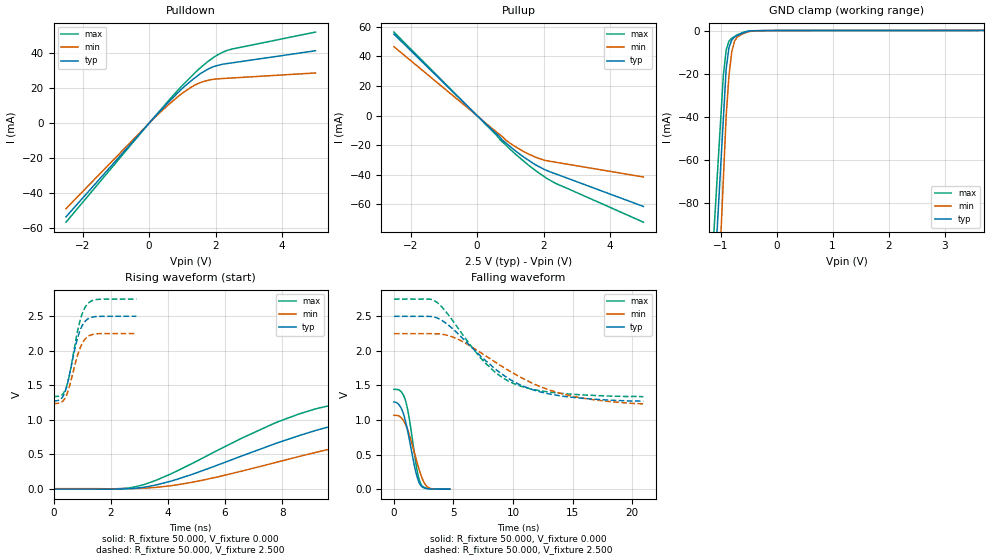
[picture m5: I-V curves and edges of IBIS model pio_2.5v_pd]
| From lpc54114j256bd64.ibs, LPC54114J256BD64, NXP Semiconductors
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[Model]   pio_2.5v_pd
Model_type I/O
Vinl=4.000E-01
Vinh=1.500E+00
Vref=0.000E+00
Rref=1.000E+06
Cref=2.000E-11
Vmeas=1.250E+00
C_comp   9.060E-12   8.700E-12   9.420E-12
[Voltage Range]   2.500E+00   2.250E+00   2.750E+00
[POWER Clamp Reference]   2.500E+00   2.250E+00   2.750E+00
[GND Clamp Reference]   0.000E+00   0.000E+00   0.000E+00
[Pullup Reference]   2.500E+00   2.250E+00   2.750E+00
[Pulldown Reference]   0.000E+00   0.000E+00   0.000E+00
[Temperature Range]   25   105   -40
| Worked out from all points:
|   slope of the pulldown table from 0 to 0.375 V, typ, clamps not added: 48.2 ohm
|   slope of the pullup table from 0 to 0.375 V, typ, clamps not added: 47.2 ohm
|   GND clamp passes 1 mA (typ) near -0.58 V on its own axis
|   rising waveform, R_fixture 50.000, V_fixture 0.000: 20-80 % time 5.59ns typ, 6.98ns min, 4.66ns max; typ from -0.006 V to 1.26 V
|   falling waveform, R_fixture 50.000, V_fixture 0.000: 20-80 % time 902ps typ, 1.09ns min, 781ps max; typ from 1.26 V to 0 V
|   rising waveform, R_fixture 50.000, V_fixture 2.500: 20-80 % time 408ps typ, 413ps min, 407ps max; typ from 1.27 V to 2.5 V
|   falling waveform, R_fixture 50.000, V_fixture 2.500: 20-80 % time 5.14ns typ, 6.37ns min, 4.26ns max; typ from 2.5 V to 1.27 V
[GND Clamp]
-2.5V     -757.5mA   -973.5mA   -687.5mA
-950mV    -40.89mA   -68.88mA   -20.67mA
-900mV    -17.78mA   -39.7mA    -9.038mA
-850mV    -7.888mA   -20.93mA   -4.915mA
-800mV    -4.357mA   -9.856mA   -3.541mA
-750mV    -3.031mA   -4.855mA   -2.756mA
-700mV    -2.227mA   -2.959mA   -1.97mA
-600mV    -1.164mA   -1.43mA    -872.3uA
-500mV    -329.3uA   -546.9uA   -245.1uA
-200mV    -21.96uA   -28.58uA   -10.55uA
5V        98.58uA    104.9uA    95.1uA
[Power Clamp]
-2.5V     0A         0A         0A
0V        0A         0A         0A
2.5V      0A         0A         0A
5V        0A         0A         0A
[Pullup]
-2.5V     55.03mA    46.51mA    56.39mA
0V        0A         0A         0A
560mV     -11.71mA   -10.66mA   -12.69mA
760mV     -16.48mA   -14.18mA   -17.72mA
1V        -20.97mA   -18.73mA   -22.83mA
1.42V     -28.23mA   -24.51mA   -31.07mA
1.96V     -35.62mA   -29.68mA   -40.25mA
2.38V     -39.45mA   -31.53mA   -45.93mA
5V        -61.32mA   -41.44mA   -71.95mA
[Pulldown]
-2.5V     -53.75mA   -49.06mA   -56.82mA
0V        0A         0A         0A
360mV     7.48mA     6.68mA     7.998mA
980mV     19.59mA    16.96mA    21.32mA
1.32V     25.16mA    21.25mA    27.81mA
1.54V     28.36mA    23.25mA    31.74mA
1.94V     32.45mA    25.18mA    37.76mA
2.36V     34.22mA    25.76mA    41.85mA
5V        41.54mA    28.79mA    52.24mA
[Rising Waveform]
R_fixture = 50.000
V_fixture = 0.000
V_fixture_min = 0.000
V_fixture_max = 0.000
|  time   V(typ)   V(min)   V(max)
0s        -5.765mV   598.8uV    -1.766mV
2.3ns     -4.275mV   340uV      -144.2uV
3.15ns    20.28mV    7.998mV    58.7mV
5ns       229.5mV    105.6mV    397.3mV
7.9ns     674.2mV    394mV      977.9mV
9.15ns    841.3mV    524.1mV    1.155V
10.4ns    976.6mV    645.3mV    1.265V
12.45ns   1.114V     810.8mV    1.354V
15.5ns    1.201V     958.7mV    1.409V
22.85ns   1.256V     1.069V     1.441V
[Falling Waveform]
R_fixture = 50.000
V_fixture = 0.000
V_fixture_min = 0.000
V_fixture_max = 0.000
|  time   V(typ)   V(min)   V(max)
0s        1.262V     1.069V     1.444V
550ps     1.189V     1.043V     1.42V
1ns       962.3mV    927.7mV    1.265V
1.3ns     714.9mV    783mV      1.01V
1.85ns    241.4mV    444.9mV    369.8mV
2.1ns     102.7mV    294.1mV    153.2mV
2.3ns     44.76mV    189.8mV    64.29mV
2.6ns     14.97mV    77.09mV    21.3mV
2.95ns    4.656mV    17.97mV    8.229mV
4.7ns     419.5uV    598.8uV    152.1uV
[Rising Waveform]
R_fixture = 50.000
V_fixture = 2.500
V_fixture_min = 2.250
V_fixture_max = 2.750
|  time   V(typ)   V(min)   V(max)
0s        1.274V     1.235V     1.337V
250ps     1.298V     1.248V     1.349V
350ps     1.353V     1.28V      1.385V
450ps     1.465V     1.352V     1.475V
600ps     1.734V     1.549V     1.738V
850ps     2.199V     1.947V     2.302V
1ns       2.363V     2.105V     2.534V
1.2ns     2.461V     2.206V     2.684V
1.55ns    2.498V     2.247V     2.745V
2.9ns     2.5V       2.25V      2.75V
[Falling Waveform]
R_fixture = 50.000
V_fixture = 2.500
V_fixture_min = 2.250
V_fixture_max = 2.750
|  time   V(typ)   V(min)   V(max)
0s        2.5V       2.25V      2.75V
2.95ns    2.499V     2.25V      2.749V
3.55ns    2.481V     2.248V     2.71V
5.25ns    2.27V      2.178V     2.363V
7.7ns     1.859V     1.929V     1.82V
8.95ns    1.68V      1.79V      1.634V
10.25ns   1.539V     1.655V     1.515V
12.25ns   1.409V     1.486V     1.425V
14.65ns   1.335V     1.357V     1.377V
20.95ns   1.274V     1.235V     1.337V
[Ramp]
dV/dt_r   7.5711E-01/5.5865E-09   6.3920E-01/6.9663E-09   8.6573E-01/4.6619E-09
dV/dt_f   7.3584E-01/5.1385E-09   6.0892E-01/6.3638E-09   8.4764E-01/4.2601E-09
R_load = 50
